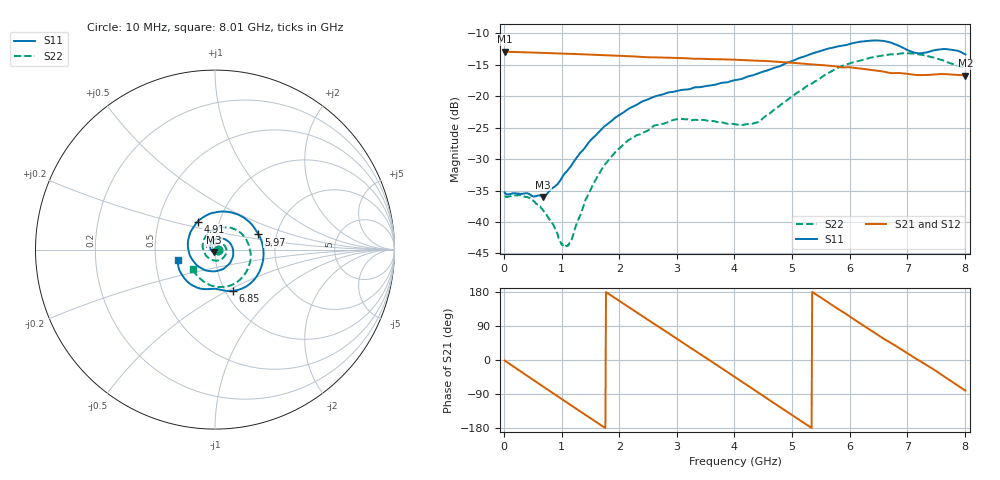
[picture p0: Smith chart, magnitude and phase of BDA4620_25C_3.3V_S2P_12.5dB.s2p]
!Agilent Technologies,E5071B,MY42404982,A.09.10
!Date: Wed May 06 08:51:09 2026
!Data & Calibration Information:
!Freq	S11:SOLT2(ON)	S21:SOLT2(ON)	S12:SOLT2(ON)	S22:SOLT2(ON)
# Hz S RI R 50
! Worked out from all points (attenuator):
!   801 points, 10 MHz to 8.01 GHz, reference 50 ohm
!   highest |S21| = -12.93 dB at 10 MHz (marker M1); lowest = -16.8 dB at 8.01 GHz (marker M2)
!   lowest |S11| = -36.0 dB at 680 MHz (marker M3), VSWR 1.03, Z = 49.6 - j1.52 ohm
!   |S11| at or under -10 dB: start of sweep to end of sweep
!   |S22| runs from -43.8 to -13.2 dB; largest |S21 - S12| = 0.0011
!   S11 on the Smith chart (normalised r, x): 10 MHz: 1.03, -0.00; 4.91 GHz: 0.79, +0.25; 5.97 GHz: 1.61, +0.29; 6.85 GHz: 1.09, -0.53; 8.01 GHz: 0.65, -0.08
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1e7  0.0172 -0.00126  0.2257 -0.00484  0.226 -0.00494  0.016 -0.000746
4.2e8  0.00906 -0.0141  0.1609 -0.1531  0.1612 -0.1534  0.0138 -0.00728
6.8e8  -0.00403 -0.0153  0.0748 -0.2073  0.0747 -0.2076  0.00755 -0.00973
1.08e9  -0.025 0.00182  -0.0778 -0.2027  -0.0779 -0.203  -0.00536 -0.00358
1.16e9  -0.0264 0.00857  -0.1053 -0.189  -0.1056 -0.1893  -0.00704 -0.000556
1.35e9  -0.0262 0.0254  -0.1607 -0.1425  -0.1608 -0.1427  -0.0093 0.00795
1.59e9  -0.0139 0.0466  -0.203 -0.0633  -0.2032 -0.0634  -0.00688 0.0205
1.9e9  0.0188 0.0628  -0.2035 0.0505  -0.2038 0.0507  0.00664 0.0339
2.31e9  0.0712 0.0473  -0.1172 0.169  -0.1174 0.1691  0.0348 0.0343
2.68e9  0.1012 -0.0031  0.00686 0.2023  0.00713 0.2025  0.0565 0.0172
3.39e9  0.0335 -0.1127  0.1888 0.0585  0.1893 0.0583  0.0458 -0.0454
4.01e9  -0.1029 -0.0853  0.1368 -0.138  0.1369 -0.1383  -0.0258 -0.054
4.41e9  -0.1508 0.0137  0.0147 -0.1899  0.0146 -0.1903  -0.0613 -0.00947
4.91e9  -0.0971 0.1557  -0.1336 -0.1279  -0.1338 -0.1282  -0.0481 0.0792
5.35e9  0.046 0.2127  -0.1783 0.000963  -0.1785 0.00101  0.0318 0.1219
5.97e9  0.2423 0.0842  -0.0804 0.1491  -0.0804 0.1493  0.1668 0.0669
6.33e9  0.2652 -0.0726  0.0224 0.1608  0.0228 0.1608  0.1985 -0.022
6.68e9  0.1707 -0.2073  0.1025 0.1137  0.1028 0.114  0.1776 -0.1178
6.85e9  0.1005 -0.2301  0.1286 0.0818  0.1289 0.0819  0.1491 -0.1569
7.18e9  0.00395 -0.2185  0.1469 0.00264  0.1472 0.00267  0.0625 -0.2063
7.54e9  -0.1007 -0.2116  0.1253 -0.0813  0.1254 -0.0813  -0.0377 -0.1937
8.01e9  -0.2065 -0.0553  0.0228 -0.1431  0.0229 -0.1435  -0.1249 -0.1088
